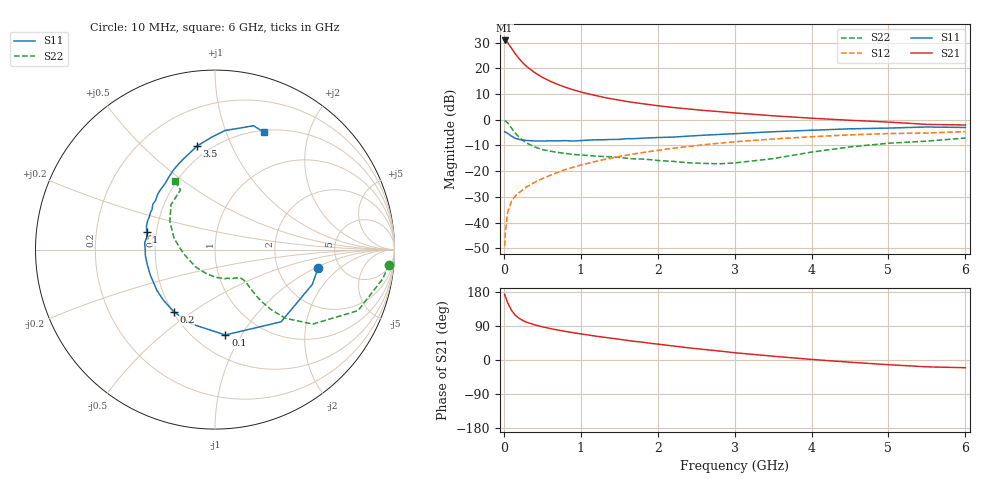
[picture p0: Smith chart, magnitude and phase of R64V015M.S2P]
! SIEMENS Small Signal Semiconductors
! BFR193
! Si NPN RF Bipolar Junction Transistor in SOT23
! VCE = 4 V  IC = 15 mA
! Common Emitter S-Parameters:  May  1996
# GHz  S  MA  R  50
!  f  S11  S21  S12  S22
! GHz  MAG  ANG  MAG  ANG  MAG  ANG  MAG  ANG
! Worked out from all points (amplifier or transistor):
!   36 points, 10 MHz to 6 GHz, reference 50 ohm
!   highest |S21| = 30.8 dB at 10 MHz (marker M1)
!   |S21| within 3 dB of that: start of sweep to 98.74 MHz
!   unconditionally stable (mu >= 1): 633.9 MHz to 1.944 GHz
!   at 250 MHz: K = 0.76, MSG = 24.6 dB, |S12| = -27.2 dB
!   at 1.4 GHz: K = 1.03, MAG = 10.5 dB, |S12| = -14.9 dB
!   at 6 GHz: K = 0.94, MSG = 1.3 dB, |S12| = -4.6 dB
!   S11 on the Smith chart (normalised r, x): 10 MHz: 3.43, -1.09; 100 MHz: 0.69, -0.85; 200 MHz: 0.51, -0.42; 1 GHz: 0.44, +0.10; 3.5 GHz: 0.43, +0.75; 6 GHz: 0.52, +1.37
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0.01  0.5835 -10.3  34.71 173.6  0.0035 84.5  0.9722 -5.0
0.02  0.5757 -19.7  34.38 167.3  0.0067 83.7  0.9485 -9.9
0.05  0.5454 -47.5  31.36 150.8  0.016 72.0  0.8665 -23.1
0.1  0.479 -83.1  24.42 131.0  0.0263 62.6  0.6849 -37.3
0.15  0.4344 -107.8  19 117.8  0.0331 60.0  0.5481 -44.3
0.2  0.4154 -123.5  15.29 109.7  0.0386 60.0  0.4548 -47.0
0.25  0.4027 -135.6  12.59 103.8  0.0439 60.4  0.3933 -48.0
0.3  0.3956 -144.8  10.73 99.4  0.05 61.7  0.3522 -48.2
0.4  0.3874 -158.4  8.277 92.9  0.0608 63.7  0.2968 -47.7
0.5  0.3863 -166.8  6.663 87.6  0.0718 65.6  0.2633 -46.8
0.6  0.3893 -174.6  5.616 83.1  0.083 66.1  0.2458 -46.4
0.7  0.3891 179.7  4.86 79.1  0.0951 66.3  0.2322 -46.8
0.8  0.3937 174.2  4.272 75.5  0.1075 66.3  0.2214 -47.4
1  0.3938 165.4  3.468 69.0  0.1315 66.0  0.2068 -49.4
1.1  0.4029 161.4  3.183 65.9  0.1438 65.1  0.202 -51.6
1.3  0.4089 153.7  2.724 60.1  0.1684 63.5  0.1927 -55.3
1.6  0.4286 143.9  2.261 51.8  0.205 60.6  0.179 -63.8
2.2  0.4601 127.4  1.732 37.1  0.2788 53.4  0.1554 -87.2
3.5  0.5851 99.9  1.194 10.0  0.4223 34.5  0.1757 -172.1
4.5  0.6663 85.1  0.977 -5.8  0.5086 20.0  0.2965 148.0
5.5  0.7229 72.7  0.813 -18.1  0.5516 5.3  0.3843 120.0
6  0.7079 67.2  0.79 -20.4  0.589 0.9  0.4417 120.5
